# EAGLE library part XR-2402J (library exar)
V.22bis high perfomance AFE
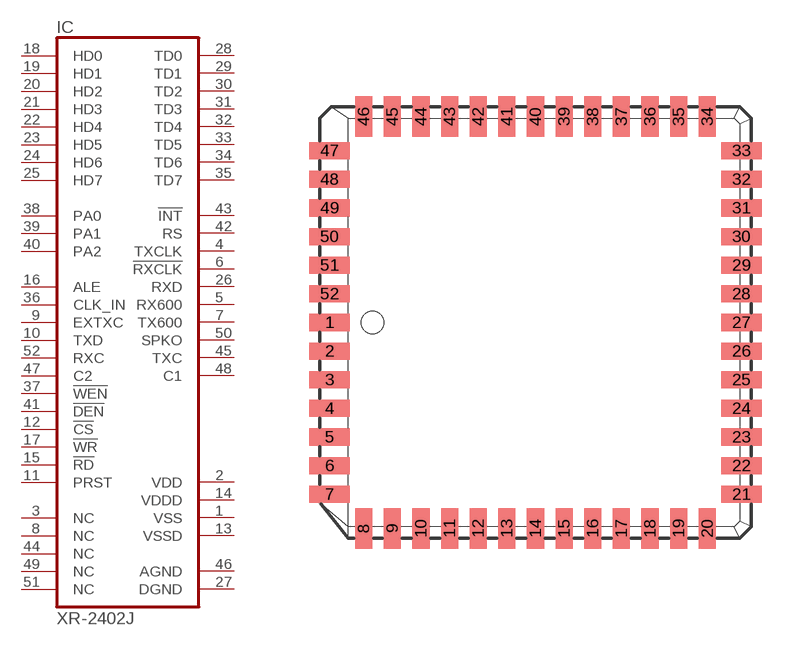
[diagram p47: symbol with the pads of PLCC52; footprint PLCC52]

Designator prefix IC

## XR-2402J (OC_FARNELL: unknown; OC_NEWARK: unknown)  [PLCC52]
1  VSS  pwr
2  VDD  pwr
3  NC  nc
4  TXCLK  out
5  RX600  out
6  !RXCLK  out
7  TX600  out
8  NC  nc
9  EXTXC  in
10  TXD  in
11  PRST  in
12  !CS  in
13  VSSD  pwr
14  VDDD  pwr
15  !RD  in
16  ALE  in
17  !WR  in
18  HD0
19  HD1
20  HD2
21  HD3
22  HD4
23  HD5
24  HD6
25  HD7
26  RXD  out
27  DGND  pwr
28  TD0
29  TD1
30  TD2
31  TD3
32  TD4
33  TD5
34  TD6
35  TD7
36  CLK_IN  in
37  !WEN  in
38  PA0  in
39  PA1  in
40  PA2  in
41  !DEN  in
42  RS  out
43  !INT  out
44  NC  nc
45  TXC  out
46  AGND  pwr
47  C2  in
48  C1  out
49  NC  nc
50  SPKO  out
51  NC  nc
52  RXC  in

## Footprint PLCC52 (pad centres in mm)
Plastic Leaded Chip Carrier
smd 1.8 x 0.76: 1 -9.13,0; 2 -9.13,-1.27; 3 -9.13,-2.54; 4 -9.13,-3.81; 5 -9.13,-5.08; 6 -9.13,-6.35; 7 -9.13,-7.62; 21 9.13,-7.62; 22 9.13,-6.35; 23 9.13,-5.08; 24 9.13,-3.81; 25 9.13,-2.54; 26 9.13,-1.27; 27 9.13,0; 28 9.13,1.27; 29 9.13,2.54; 30 9.13,3.81; 31 9.13,5.08; 32 9.13,6.35; 33 9.13,7.62; 47 -9.13,7.62; 48 -9.13,6.35; 49 -9.13,5.08; 50 -9.13,3.81; 51 -9.13,2.54; 52 -9.13,1.27
smd 0.76 x 1.8: 8 -7.62,-9.13; 9 -6.35,-9.13; 10 -5.08,-9.13; 11 -3.81,-9.13; 12 -2.54,-9.13; 13 -1.27,-9.13; 14 0,-9.13; 15 1.27,-9.13; 16 2.54,-9.13; 17 3.81,-9.13; 18 5.08,-9.13; 19 6.35,-9.13; 20 7.62,-9.13; 34 7.62,9.13; 35 6.35,9.13; 36 5.08,9.13; 37 3.81,9.13; 38 2.54,9.13; 39 1.27,9.13; 40 0,9.13; 41 -1.27,9.13; 42 -2.54,9.13; 43 -3.81,9.13; 44 -5.08,9.13; 45 -6.35,9.13; 46 -7.62,9.13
